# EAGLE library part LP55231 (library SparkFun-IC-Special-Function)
LP55231 Programmable 9-Output LED Driver Datasheet SparkFun Products: SparkFun LED Driver Breakout - LP55231
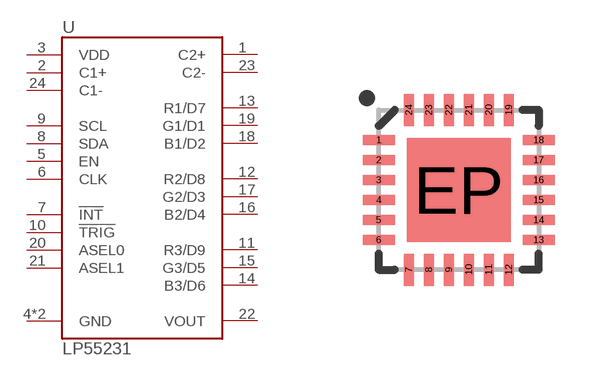
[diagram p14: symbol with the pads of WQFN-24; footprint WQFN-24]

Designator prefix U

## LP55231WQFN (PROD_ID: IC-13302)  [WQFN-24]
1  C2+
2  C1+
3  VDD
4  GND
5  EN
6  CLK
7  !INT
8  SDA
9  SCL
10  !TRIG
11  R3/D9
12  R2/D8
13  R1/D7
14  B3/D6
15  G3/D5
16  B2/D4
17  G2/D3
18  B1/D2
19  G1/D1
20  ASEL0
21  ASEL1
22  VOUT
23  C2-
24  C1-
EP  GND

## Footprint WQFN-24 (pad centres in mm)
WQFN - 24 Pin Specifications: Pin count: 24 Datasheet referenced for footprint Example device(s): LP55231
smd 0.8 x 0.25: 1 -2,1.25; 2 -2,0.75; 3 -2,0.25; 4 -2,-0.25; 5 -2,-0.75; 6 -2,-1.25; 13 2,-1.25; 14 2,-0.75; 15 2,-0.25; 16 2,0.25; 17 2,0.75; 18 2,1.25
smd 0.25 x 0.8: 7 -1.25,-2; 8 -0.75,-2; 9 -0.25,-2; 10 0.25,-2; 11 0.75,-2; 12 1.25,-2; 19 1.25,2; 20 0.75,2; 21 0.25,2; 22 -0.25,2; 23 -0.75,2; 24 -1.25,2
smd 2.6 x 2.6: EP 0,0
